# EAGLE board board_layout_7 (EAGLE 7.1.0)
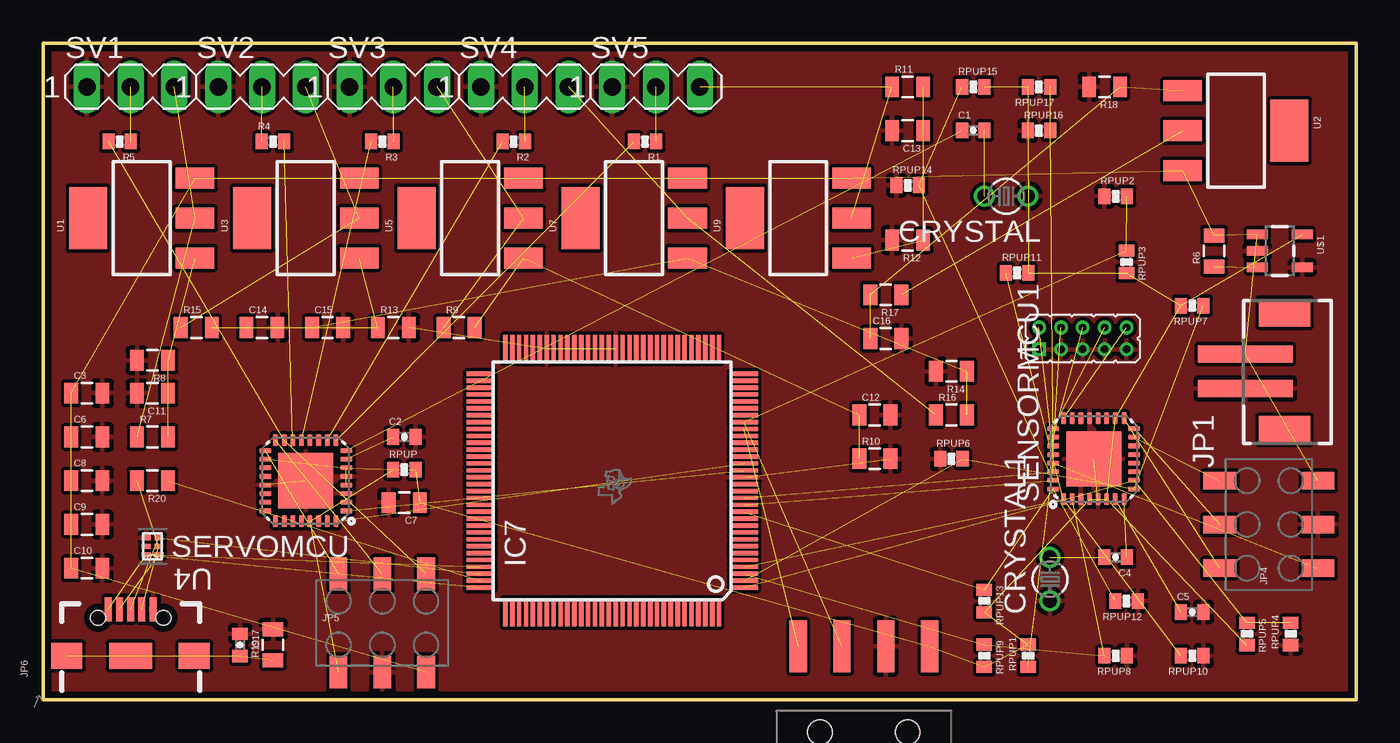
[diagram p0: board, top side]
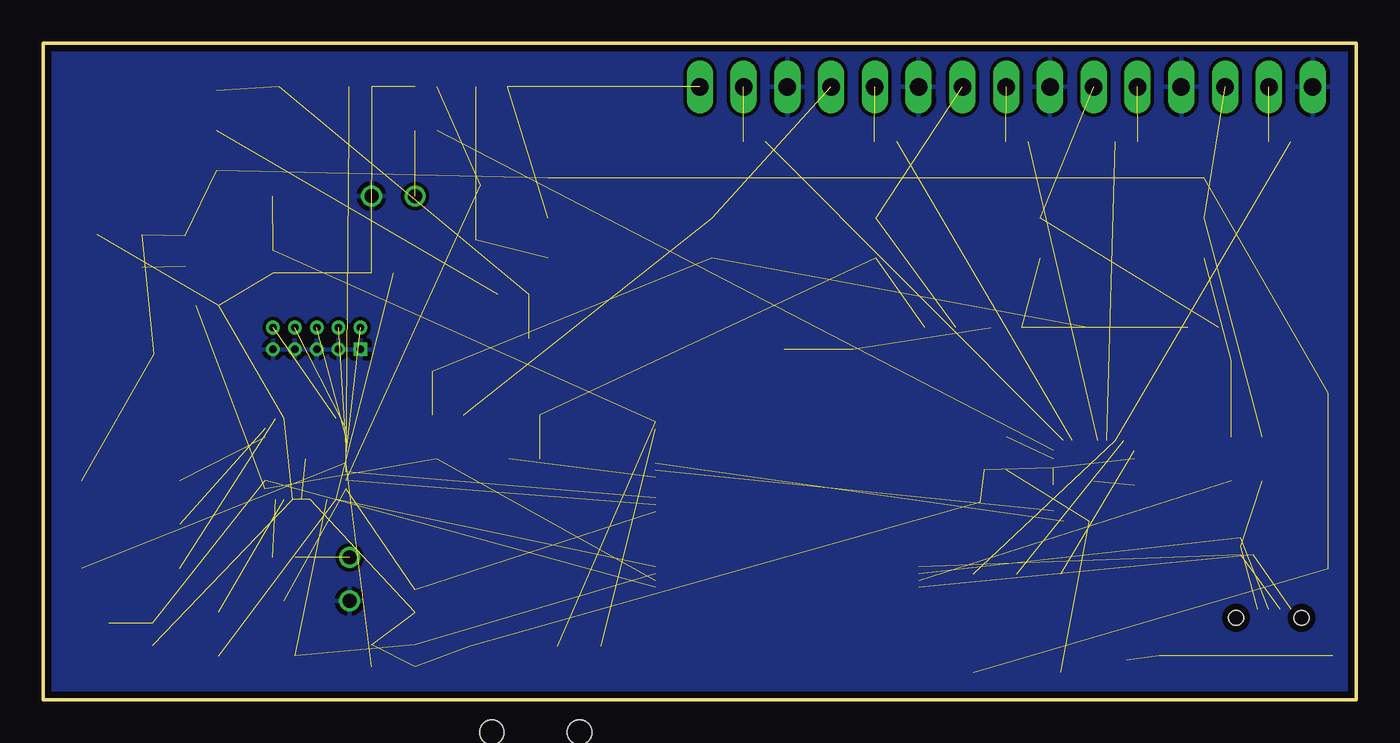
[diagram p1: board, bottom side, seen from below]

Size 76.2 x 38.1 mm. Coordinates in mm from the lower left corner, seen from the top.
Outline: 0,0 0,38.1 76.2,38.1 76.2,0 0,0
Copper layers (1*16): Top 0.0356mm / dielectric 1.5011mm / Bottom 0.0356mm
Design rules "LaenPCBOrder": minimum track width 6mil, minimum drill 13mil, track to track 6mil, track to pad 6mil, pad to pad 6mil, via to via 6mil, smd to smd 6mil, copper to edge 15mil, drill to drill 6mil, minimum pad ring 7mil, minimum via ring 7mil, stop-mask expansion 3mil, vias tented up to drill 0mil, thermal gap 10mil
Net classes: 0 default: clearance 0.205 mm

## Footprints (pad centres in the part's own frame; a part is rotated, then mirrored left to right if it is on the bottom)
0402-CAP = smd 0.7 x 0.9: 1 -0.65,0; 2 0.65,0
0805 = smd 0.8 x 1.2: 1 -0.9,0; 2 0.9,0
TC26V = drill 0.813: 1 -1.27,0; 2 1.27,0
PDT_S-PQFP-G128 = smd 0.25 x 1.6: 1 -6.2,-7.65; 2 -5.8,-7.65; 3 -5.4,-7.65; 4 -5,-7.65; 5 -4.6,-7.65; 6 -4.2,-7.65; 7 -3.8,-7.65; 8 -3.4,-7.65; 9 -3,-7.65; 10 -2.6,-7.65; 11 -2.2,-7.65; 12 -1.8,-7.65; 13 -1.4,-7.65; 14 -1,-7.65; 15 -0.6,-7.65; 16 -0.2,-7.65; 17 0.2,-7.65; 18 0.6,-7.65; 19 1,-7.65; 20 1.4,-7.65; 21 1.8,-7.65; 22 2.2,-7.65; 23 2.6,-7.65; 24 3,-7.65; 25 3.4,-7.65; 26 3.8,-7.65; 27 4.2,-7.65; 28 4.6,-7.65; 29 5,-7.65; 30 5.4,-7.65; 31 5.8,-7.65; 32 6.2,-7.65; 65 6.2,7.65; 66 5.8,7.65; 67 5.4,7.65; 68 5,7.65; 69 4.6,7.65; 70 4.2,7.65; 71 3.8,7.65; 72 3.4,7.65; 73 3,7.65; 74 2.6,7.65; 75 2.2,7.65; 76 1.8,7.65; 77 1.4,7.65; 78 1,7.65; 79 0.6,7.65; 80 0.2,7.65; 81 -0.2,7.65; 82 -0.6,7.65; 83 -1,7.65; 84 -1.4,7.65; 85 -1.8,7.65; 86 -2.2,7.65; 87 -2.6,7.65; 88 -3,7.65; 89 -3.4,7.65; 90 -3.8,7.65; 91 -4.2,7.65; 92 -4.6,7.65; 93 -5,7.65; 94 -5.4,7.65; 95 -5.8,7.65; 96 -6.2,7.65 | smd 1.6 x 0.25: 33 7.65,-6.2; 34 7.65,-5.8; 35 7.65,-5.4; 36 7.65,-5; 37 7.65,-4.6; 38 7.65,-4.2; 39 7.65,-3.8; 40 7.65,-3.4; 41 7.65,-3; 42 7.65,-2.6; 43 7.65,-2.2; 44 7.65,-1.8; 45 7.65,-1.4; 46 7.65,-1; 47 7.65,-0.6; 48 7.65,-0.2; 49 7.65,0.2; 50 7.65,0.6; 51 7.65,1; 52 7.65,1.4; 53 7.65,1.8; 54 7.65,2.2; 55 7.65,2.6; 56 7.65,3; 57 7.65,3.4; 58 7.65,3.8; 59 7.65,4.2; 60 7.65,4.6; 61 7.65,5; 62 7.65,5.4; 63 7.65,5.8; 64 7.65,6.2; 97 -7.65,6.2; 98 -7.65,5.8; 99 -7.65,5.4; 100 -7.65,5; 101 -7.65,4.6; 102 -7.65,4.2; 103 -7.65,3.8; 104 -7.65,3.4; 105 -7.65,3; 106 -7.65,2.6; 107 -7.65,2.2; 108 -7.65,1.8; 109 -7.65,1.4; 110 -7.65,1; 111 -7.65,0.6; 112 -7.65,0.2; 113 -7.65,-0.2; 114 -7.65,-0.6; 115 -7.65,-1; 116 -7.65,-1.4; 117 -7.65,-1.8; 118 -7.65,-2.2; 119 -7.65,-2.6; 120 -7.65,-3; 121 -7.65,-3.4; 122 -7.65,-3.8; 123 -7.65,-4.2; 124 -7.65,-4.6; 125 -7.65,-5; 126 -7.65,-5.4; 127 -7.65,-5.8; 128 -7.65,-6.2
JST-2-SMD-VERT = smd 1 x 5.5: GND 1,-2; VCC -1,-2 | smd 1.6 x 3: P$1 -3.4,0.27; P$2 3.4,0.27
2X5_PTH_SILK_.05 = drill 0.432 square: 1 0,6.35 | drill 0.432: 2 1.27,6.35; 3 0,5.08; 4 1.27,5.08; 5 0,3.81; 6 1.27,3.81; 7 0,2.54; 8 1.27,2.54; 9 0,1.27; 10 1.27,1.27
1X04-SMD = smd 1 x 3: 1 -3.81,5; 2 -1.27,5; 3 1.27,5; 4 3.81,5 | hole 1.4: -2.54,0; 2.54,0
2X3_SMD = smd 1.02 x 1.9: 1 -2.54,-2.85; 2 -2.54,2.85; 3 0,-2.85; 4 0,2.85; 5 2.54,-2.85; 6 2.54,2.85
USB-B-MICRO-SMD_V03 = smd 1.4 x 0.4: D+1 2.7,0; D-1 2.7,0.65; GND1 2.7,-1.3; ID1 2.7,-0.65; VBUS1 2.7,1.3 | smd 1.5 x 1.8: SHIELD1 0,3.7; SHIELD2 0,-3.7 | smd 1.5 x 2.5: SHIELD3 0,0 | hole 0.85: 2.2,1.9; 2.2,-1.9
0402-RES = smd 0.7 x 0.9: 1 -0.65,0; 2 0.65,0
MLF32-PAD = smd 0.7 x 0.3: 1 -2.35,1.75; 2 -2.35,1.25; 3 -2.35,0.75; 4 -2.35,0.25; 5 -2.35,-0.25; 6 -2.35,-0.75; 7 -2.35,-1.25; 8 -2.35,-1.75; 17 2.35,-1.75; 18 2.35,-1.25; 19 2.35,-0.75; 20 2.35,-0.25; 21 2.35,0.25; 22 2.35,0.75; 23 2.35,1.25; 24 2.35,1.75 | smd 0.3 x 0.7: 9 -1.75,-2.35; 10 -1.25,-2.35; 11 -0.75,-2.35; 12 -0.25,-2.35; 13 0.25,-2.35; 14 0.75,-2.35; 15 1.25,-2.35; 16 1.75,-2.35; 25 1.75,2.35; 26 1.25,2.35; 27 0.75,2.35; 28 0.25,2.35; 29 -0.25,2.35; 30 -0.75,2.35; 31 -1.25,2.35; 32 -1.75,2.35 | smd 3.2 x 3.2: PAD 0,0
MA03-1 = drill 1.016 long: 1 -2.54,0; 2 0,0; 3 2.54,0
SOT223 = smd 1.219 x 2.235: 1 -2.311,-3.099; 2 0,-3.099; 3 2.311,-3.099 | smd 3.6 x 2.2: 4 0,3.099
DRY6 = smd 0.559 x 0.305: 1 -0.355,0.5 | smd 0.508 x 0.305: 2 -0.37,0; 3 -0.37,-0.5; 4 0.37,-0.5; 5 0.37,0; 6 0.37,0.5
SOT23-5 = smd 0.55 x 1.2: 1 -0.95,-1.3; 2 0,-1.3; 3 0.95,-1.3; 4 0.95,1.3; 5 -0.95,1.3

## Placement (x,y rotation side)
C1  22pf  [0402-CAP]  53.98,33.02 0 top
C2  22pf  [0402-CAP]  20.95,15.24 0 top
C3  10uF  [0805]  2.54,17.78 0 top
C4  22pf  [0402-CAP]  62.23,8.26 180 top
C5  22pf  [0402-CAP]  66.67,5.08 0 top
C6  0.1 uF  [0805]  2.54,15.24 0 top
C7  0.47 uF  [0805]  20.95,11.43 180 top
C8  2200uF  [0805]  2.54,12.7 0 top
C9  100nF  [0805]  2.54,10.16 0 top
C10  100nF  [0805]  2.54,7.62 0 top
C11  10uF  [0805]  6.35,17.78 180 top
C12  10uF  [0805]  48.26,16.51 0 top
C13  10uF  [0805]  50.16,33.02 180 top
C14  10uF  [0805]  12.7,21.59 0 top
C15  10uF  [0805]  16.51,21.59 0 top
C16  10uF  [0805]  48.9,20.95 0 top
C17  3300pf  [0402-CAP]  11.43,3.17 270 top
CRYSTAL  16MHz  [TC26V]  55.88,29.21 180 top
CRYSTAL1  16MHz  [TC26V]  58.42,6.99 90 top
IC7  TM4C129XXXPDT  [PDT_S-PQFP-G128]  33.02,12.7 90 top
JP1  M024UCON-15767  [JST-2-SMD-VERT]  71.75,19.05 270 top
JP2  M05X20.05_IN_PTH_SILK  [2X5_PTH_SILK_.05]  64.14,20.32 90 top
JP3  [1X04-SMD]  47.62,-1.91 0 top
JP4  [2X3_SMD]  71.12,10.16 90 top
JP5  [2X3_SMD]  19.68,4.45 0 top
JP6  USB_MICROB_PLUGCONN-11752  [USB-B-MICRO-SMD_V03]  5.08,2.54 90 top
R1  1k  [0402-RES]  34.92,32.38 180 top
R2  1k  [0402-RES]  27.3,32.38 180 top
R3  1k  [0402-RES]  19.68,32.38 180 top
R4  1k  [0402-RES]  13.34,32.38 0 top
R5  1k  [0402-RES]  4.45,32.38 180 top
R6  10k  [0805]  67.94,26.04 90 top
R7  220  [0805]  6.35,15.24 0 top
R8  820  [0805]  6.35,19.68 180 top
R9  220  [0805]  24.13,21.59 0 top
R10  820  [0805]  48.26,13.97 0 top
R11  220  [0805]  50.16,35.56 0 top
R12  820  [0805]  50.16,26.67 180 top
R13  820  [0805]  20.32,21.59 0 top
R14  820  [0805]  52.7,19.05 180 top
R15  220  [0805]  8.89,21.59 0 top
R16  220  [0805]  52.7,16.51 0 top
R17  220  [0805]  48.9,23.5 180 top
R18  360  [0805]  61.59,35.56 180 top
R19  1M  [0805]  13.34,3.17 90 top
R20  100  [0805]  6.35,12.7 180 top
RPUP  10k  [0402-RES]  20.95,13.34 0 top
RPUP1  10k  [0402-RES]  57.15,2.54 90 top
RPUP2  680  [0402-RES]  62.23,29.21 0 top
RPUP3  330  [0402-RES]  62.87,25.4 270 top
RPUP4  680  [0402-RES]  72.39,3.81 90 top
RPUP5  330  [0402-RES]  69.85,3.81 270 top
RPUP6  680  [0402-RES]  52.7,13.97 0 top
RPUP7  330  [0402-RES]  66.67,22.86 180 top
RPUP8  680  [0402-RES]  62.23,2.54 180 top
RPUP9  330  [0402-RES]  54.61,2.54 270 top
RPUP10  680  [0402-RES]  66.67,2.54 180 top
RPUP11  330  [0402-RES]  56.52,24.77 0 top
RPUP12  680  [0402-RES]  62.87,5.71 180 top
RPUP13  330  [0402-RES]  54.61,5.71 270 top
RPUP14  680  [0402-RES]  50.16,29.84 0 top
RPUP15  330  [0402-RES]  53.98,35.56 0 top
RPUP16  680  [0402-RES]  57.78,33.02 0 top
RPUP17  330  [0402-RES]  57.78,35.56 180 top
SENSORMCU1  atmega328p  [MLF32-PAD]  60.96,13.97 90 top
SERVOMCU  atmega328p  [MLF32-PAD]  15.24,12.7 180 top
SV1  sv1  [MA03-1]  5.08,35.56 0 top
SV2  sv2  [MA03-1]  12.7,35.56 0 top
SV3  sv3  [MA03-1]  20.32,35.56 0 top
SV4  sv4  [MA03-1]  27.94,35.56 0 top
SV5  sv5  [MA03-1]  35.56,35.56 0 top
U1  V_REG_317SMD  [SOT223]  5.71,27.94 90 top
U2  V_REG_317SMD  [SOT223]  69.22,33.02 270 top
U3  V_REG_317SMD  [SOT223]  15.24,27.94 90 top
U4  TPD4S012_DRY_6  [DRY6]  6.35,8.89 180 top
U5  V_REG_317SMD  [SOT223]  24.77,27.94 90 top
U7  V_REG_317SMD  [SOT223]  34.29,27.94 90 top
U9  V_REG_317SMD  [SOT223]  43.81,27.94 90 top
U$1  5V  [SOT23-5]  71.75,26.04 270 top

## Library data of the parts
C1 C2 C4-C7 C17 R1-R20 RPUP RPUP1-RPUP17 = SparkFun-Passives
C3 C8-C16 = SparkFun-Capacitors
CRYSTAL CRYSTAL1 = crystal; OC_FARNELL: unknown; OC_NEWARK: unknown
IC7 = ti-tiva
JP1-JP3 = SparkFun-Connectors
JP4 JP5 = SparkFun-Connectors; PROD_ID: CONN-11290
JP6 = SparkFun-Connectors; PROD_ID: CONN-11752
SENSORMCU1 SERVOMCU = SparkFun-DigitalIC
SV1-SV5 = con-lstb; OC_FARNELL: unknown; OC_NEWARK: unknown
U1-U3 U5 U7 U9 = SparkFun-PowerIC
U4 = esd_tp; DATASHEETURL: http://www.ti.com/lit/gpn/TPD4S012; DESCRIPTION: 4-Channel USB ESD Solution with Power Clamp; FAMILY_NAME: ESD Solution; GENERIC_PART_NUMBER: TPD4S012; INDUSTRY_STD_PKG_TYPE: SON; MANUFACTURER: Texas Instruments; MANUFACTURER_PART_NUMBER: tpd4s012_dry_6; PACKAGE_DESIGNATOR: DRY; PIN_COUNT: 6; VENDOR: Texas Instruments
U$1 = SparkFun-PowerIC; PROD_ID: VREG-00823

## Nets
3.3V: R17.1 U2.2
5.0V: C7.1 JP3.4 RPUP1.2 RPUP3.2 RPUP5.2 RPUP7.2 RPUP9.2 RPUP11.2 RPUP13.2 RPUP15.2 RPUP17.2 RPUP.2 SENSORMCU1.4 SENSORMCU1.6 SENSORMCU1.18 SERVOMCU.4 SERVOMCU.6 SERVOMCU.18 U$1.5
A2T1: IC7.1 RPUP4.2 RPUP5.1 SENSORMCU1.10
A2T2: IC7.2 RPUP6.2 RPUP7.1 SENSORMCU1.9
A2T3: IC7.3 RPUP8.2 RPUP9.1 SENSORMCU1.2
A2T4: IC7.4 RPUP10.2 RPUP11.1 SENSORMCU1.1
A2T5: IC7.12 RPUP12.2 RPUP13.1 SENSORMCU1.32
A2T6: IC7.13 RPUP14.2 RPUP15.1 SENSORMCU1.31
A2T7: IC7.14 RPUP16.2 RPUP17.1 SENSORMCU1.30
GND: C2.2 C3.2 C5.2 C6.2 C7.2 C8.2 C9.2 C10.2 C11.2 C12.2 C13.2 C14.2 C15.2 C16.2 C17.1 CRYSTAL1.1 CRYSTAL.1 IC7.17 IC7.48 IC7.58 JP1.GND JP2.1 JP2.3 JP2.5 JP2.7 JP2.9 JP3.3 JP4.3 JP5.3 JP6.GND1 R8.2 R10.2 R12.2 R13.2 R14.2 R18.2 R19.2 RPUP2.1 RPUP4.1 RPUP6.1 RPUP8.1 RPUP10.1 RPUP12.1 RPUP14.1 RPUP16.1 SENSORMCU1.3 SENSORMCU1.5 SENSORMCU1.21 SENSORMCU1.PAD SERVOMCU.3 SERVOMCU.5 SERVOMCU.21 SERVOMCU.PAD SV1.1 SV2.1 SV3.1 SV4.1 SV5.1 U4.4 U$1.2 U$1.4
MISO: JP4.4 SENSORMCU1.16
MISO1: JP5.4 SERVOMCU.16
MOSI: JP4.6 SENSORMCU1.15
MOSI1: JP5.6 R5.2 SERVOMCU.15
N$1: R6.1 U$1.3
N$2: R4.2 SERVOMCU.14
N$3: R3.2 SERVOMCU.13
N$4: C11.1 R7.2 R8.1 U1.1
N$5: R2.1 SV4.2
N$6: R1.1 SV5.2
N$7: R2.2 SERVOMCU.10
N$8: R1.2 SERVOMCU.9
N$9: R3.1 SV3.2
N$10: C1.1 SERVOMCU.8
N$11: C2.1 SERVOMCU.7
N$12: R5.1 SV1.2
N$13: R4.1 SV2.2
N$14: C16.1 R17.2 R18.1 U2.1
N$15: JP2.10 SENSORMCU1.24
N$16: JP2.8 SENSORMCU1.25
N$17: C4.1 SENSORMCU1.8
N$18: C4.2 CRYSTAL1.2
N$19: C5.1 SENSORMCU1.7
N$20: C1.2 CRYSTAL.2
N$21: JP2.6 SENSORMCU1.26
N$22: JP2.4 SENSORMCU1.27
N$23: JP2.2 SENSORMCU1.28
N$24: IC7.80
N$25: C12.1 R9.2 R10.1 U5.1
N$26: C13.1 R11.2 R12.1 U9.1
N$27: IC7.114
N$28: IC7.90
N$29: C14.1 R13.1 R15.2 U3.1
N$30: IC7.87
N$31: C15.1 R14.1 R16.2 U7.1
N$32: IC7.113
N$33: IC7.122
N$38: C17.2 JP6.SHIELD1 JP6.SHIELD2 JP6.SHIELD3 R19.1
PB0/3.2C: IC7.95 R20.1
PK0_RX: IC7.18 SERVOMCU.1
PK1_TX: IC7.19 SERVOMCU.32
RESET: JP4.1 RPUP1.1 SENSORMCU1.29
RESET1: JP5.1 RPUP.1 SERVOMCU.29
RX_HC: IC7.24 JP3.1
SCK: JP4.2 SENSORMCU1.17
SCK1: JP5.2 SERVOMCU.17
SV1PS: R7.1 SV1.3 U1.2
SV2PS: R15.1 SV2.3 U3.2
SV3PS: R9.1 SV3.3 U5.2
SV4PS: R16.1 SV4.3 U7.2
SV5PS: R11.1 SV5.3 U9.2
TARGET_ID: JP6.ID1 R20.2 U4.2
TARGET_VBUS/3.2C: IC7.96 JP6.VBUS1 U4.6
TX_HC: IC7.25 JP3.2 RPUP2.2 RPUP3.1
USBD_N: IC7.93 JP6.D-1 U4.1
USBD_P: IC7.94 JP6.D+1 U4.3
VCC: C3.1 C6.1 C8.1 C9.1 C10.1 JP1.VCC JP4.5 JP5.5 R6.2 U1.3 U2.3 U3.3 U5.3 U7.3 U9.3 U$1.1

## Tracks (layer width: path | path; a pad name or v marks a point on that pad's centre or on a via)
3.3V  (1 unrouted)
5.0V  (18 unrouted)
A2T1  (3 unrouted)
A2T2  (3 unrouted)
A2T3  (3 unrouted)
A2T4  (3 unrouted)
A2T5  (3 unrouted)
A2T6  (3 unrouted)
A2T7  (3 unrouted)
GND  (5 unrouted)
  pour Top (isolate 0.152): 0,38.1 76.2,38.1 76.2,0 0,0
  pour Bottom (isolate 0.152): 0,38.1 76.2,38.1 76.2,0 0,0
MISO  (1 unrouted)
MISO1  (1 unrouted)
MOSI  (1 unrouted)
MOSI1  (2 unrouted)
N$1  (1 unrouted)
N$2  (1 unrouted)
N$3  (1 unrouted)
N$4  (3 unrouted)
N$5  (1 unrouted)
N$6  (1 unrouted)
N$7  (1 unrouted)
N$8  (1 unrouted)
N$9  (1 unrouted)
N$10  (1 unrouted)
N$11  (1 unrouted)
N$12  (1 unrouted)
N$13  (1 unrouted)
N$14  (3 unrouted)
N$15  (1 unrouted)
N$16  (1 unrouted)
N$17  (1 unrouted)
N$18  (1 unrouted)
N$19  (1 unrouted)
N$20  (1 unrouted)
N$21  (1 unrouted)
N$22  (1 unrouted)
N$23  (1 unrouted)
N$25  (3 unrouted)
N$26  (3 unrouted)
N$29  (3 unrouted)
N$31  (3 unrouted)
N$38  (4 unrouted)
PB0/3.2C  (1 unrouted)
PK0_RX  (1 unrouted)
PK1_TX  (1 unrouted)
RESET  (2 unrouted)
RESET1  (2 unrouted)
RX_HC  (1 unrouted)
SCK  (1 unrouted)
SCK1  (1 unrouted)
SV1PS  (2 unrouted)
SV2PS  (2 unrouted)
SV3PS  (2 unrouted)
SV4PS  (2 unrouted)
SV5PS  (2 unrouted)
TARGET_ID  (2 unrouted)
TARGET_VBUS/3.2C  (2 unrouted)
TX_HC  (3 unrouted)
USBD_N  (2 unrouted)
USBD_P  (2 unrouted)
VCC  (15 unrouted)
